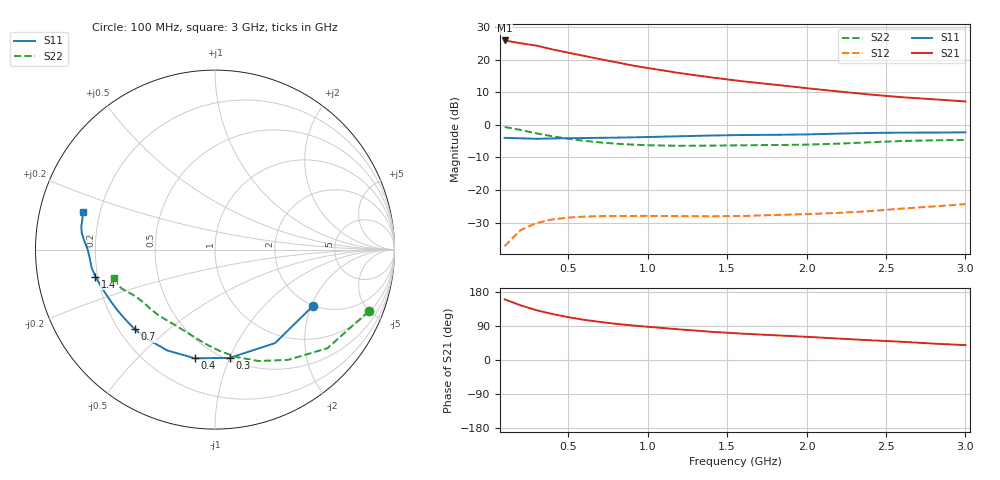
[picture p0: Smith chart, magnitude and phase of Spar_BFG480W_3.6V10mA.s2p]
! Filename: 3_610BFG480.001
! Title: BFG480W
! Bias: Vce=3.6V; Ic=10mA
! Company: NXP Semiconductors NL
! User: Quality&Reliability T&D
! Measure time: 10 Nov 1999 / 11:59:12
#  MHz  S  MA  R 50
! Freq  S11  S21  S12  S22  :
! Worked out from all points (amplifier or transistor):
!   20 points, 100 MHz to 3 GHz, reference 50 ohm
!   highest |S21| = 25.9 dB at 100 MHz (marker M1)
!   |S21| within 3 dB of that: start of sweep to 426.4 MHz
!   unconditionally stable (mu >= 1): 1.682 GHz to end of sweep
!   at 400 MHz: K = 0.24, MSG = 26.1 dB, |S12| = -29.1 dB
!   at 1.2 GHz: K = 0.73, MSG = 22.0 dB, |S12| = -28.0 dB
!   at 3 GHz: K = 1.16, MAG = 13.4 dB, |S12| = -24.4 dB
!   S11 on the Smith chart (normalised r, x): 100 MHz: 2.00, -2.07; 300 MHz: 0.52, -1.00; 400 MHz: 0.39, -0.76; 700 MHz: 0.26, -0.39; 1.4 GHz: 0.19, -0.11; 3 GHz: 0.14, +0.14
100  0.6301 -29.7  19.63 160.1  0.0137 69.1  0.9229 -21.9
200  0.6191 -57.3  17.81 144.4  0.02414 56.9  0.833 -41.3
300  0.6087 -82.3  16.35 131.5  0.03098 47.6  0.7372 -56.4
400  0.6158 -100.4  14.33 121.4  0.03524 40.6  0.6661 -68.7
500  0.6216 -115.2  12.75 113.1  0.03756 35.8  0.6091 -79.0
600  0.6247 -126.8  11.39 106.0  0.03893 32.7  0.5665 -87.1
700  0.6299 -135.4  10.15 100.4  0.03956 30.6  0.5355 -93.9
800  0.6337 -142.6  9.114 95.5  0.03979 29.5  0.5122 -99.8
900  0.64 -148.0  8.151 91.4  0.03985 29.3  0.496 -105.0
1000  0.6475 -153.2  7.418 87.7  0.03996 29.5  0.4846 -110.1
1200  0.6655 -161.4  6.212 80.8  0.03961 30.8  0.4754 -118.9
1400  0.6832 -167.3  5.322 74.4  0.03929 33.5  0.4781 -126.2
1600  0.6953 -171.9  4.635 69.5  0.03984 37.8  0.4836 -132.0
1800  0.7 -176.3  4.117 65.3  0.04125 42.8  0.4882 -137.6
2000  0.7101 179.8  3.637 61.2  0.04254 47.9  0.495 -143.4
2200  0.7308 176.0  3.245 56.6  0.04442 52.0  0.5123 -149.2
2400  0.748 172.9  2.906 52.1  0.04726 55.7  0.5383 -153.9
2600  0.756 170.2  2.644 48.1  0.05172 59.0  0.5625 -157.2
2800  0.7578 167.3  2.459 43.2  0.05577 60.8  0.5765 -160.3
3000  0.7642 164.0  2.275 39.3  0.0605 62.7  0.586 -164.2
